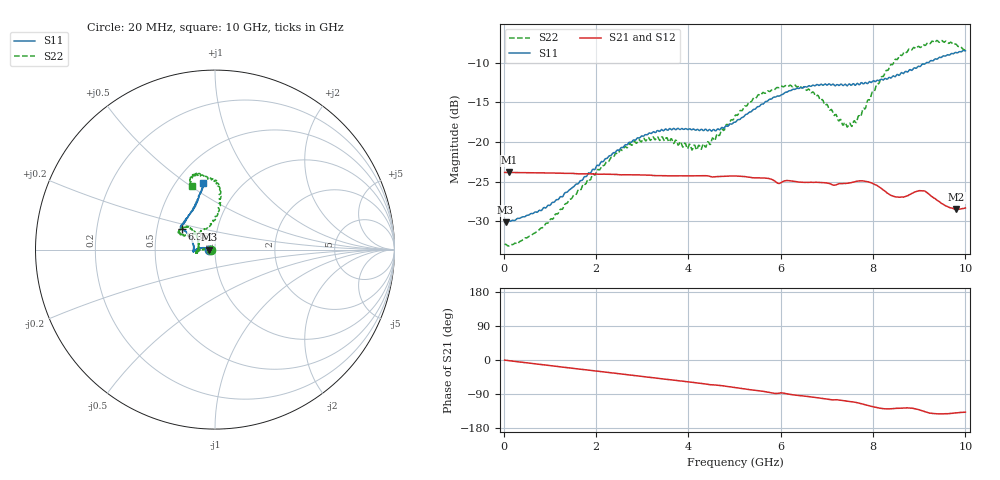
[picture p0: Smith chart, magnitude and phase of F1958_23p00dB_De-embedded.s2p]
! Integrated Device Technology
! Corporate Headquarters
! 6024 Silver Creek Valley Road
! San Jose, CA 95138  USA
! Phone:  1-408-284-8200
! Toll Free:  1-800-223-1366
! Webpage:  http://www.idt.com/
! Timing and RF Division
! 515 Groton Road, Suite 102
! Westford, MA 01886-6024
! Device:  F1958
! Description: 7-bit 0.25 dB Digital Step Attenuator
! Frequency:  0.001 -  6.000 GHz
! Package:  4x4 mm Thin QFN Plastic Package: 24 pin
! Ports:  2 RF, 12 DC
!  Pin  1  = D0
!  Pin  2  = VDD
!  Pin  3  = VMODE
!  Pin  4  = GND
!  Pin  5  = RF1  =  Port 1
!  Pin  6  = GND
!  Pin  7  = GND
!  Pin  8  = GND
!  Pin  9  = GND
!  Pin 10  = GND
!  Pin 11  = GND
!  Pin 12  = GND
!  Pin 13  = GND
!  Pin 14  = RF2  =  Port 2
!  Pin 15  = GND
!  Pin 16  = LE
!  Pin 17  = CLK
!  Pin 18  = DATA
!  Pin 19  = D6
!  Pin 20  = D5
!  Pin 21  = D4
!  Pin 22  = D3
!  Pin 23  = D2
!  Pin 24  = D1
! State:  92
! Atten State:  23.00 dB
! Voltage:  +3.30 Volts
! Current:  0.258 mA
! Data:  The device was measured on a F1958 evaluation board which has
!  individual transmission lines to the RF pins.  Data was collected
!  using a calibrated network analyzer.  The evaluation board was
!  de-embedded using Automatic Fixture Removal (AFR).
!  The reference plane is the edge of the package pin.
! Misc:
!  Action Tracker AT0419
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# GHz S dB R 50
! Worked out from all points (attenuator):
!   500 points, 20 MHz to 10 GHz, reference 50 ohm
!   highest |S21| = -23.84 dB at 120 MHz (marker M1); lowest = -28.5 dB at 9.8 GHz (marker M2)
!   lowest |S11| = -30.1 dB at 40 MHz (marker M3), VSWR 1.06, Z = 47 - j0.0425 ohm
!   |S11| at or under -10 dB: start of sweep to 9.151 GHz
!   |S22| runs from -33.2 to -7.2 dB; largest |S21 - S12| = 0.00036
!   S11 on the Smith chart (normalised r, x): 20 MHz: 0.94, -0.00; 6.36 GHz: 0.67, +0.16; 10 GHz: 0.67, +0.58
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0.02  -30.10 -179.0  -23.85 -0.3  -23.84 -0.3  -32.97 -178.3
0.04  -30.12 -179.2  -23.84 -0.6  -23.84 -0.6  -32.91 -177.5
0.12  -30.01 178.8  -23.84 -1.8  -23.84 -1.8  -33.09 -179.5
0.84  -28.50 170.7  -23.91 -12.4  -23.90 -12.4  -30.83 178.4
1.7  -24.84 170.7  -24.02 -24.7  -24.02 -24.6  -25.62 177.3
2.6  -20.61 176.7  -24.14 -37.6  -24.12 -37.6  -20.83 -177.3
3.36  -18.65 -175.7  -24.25 -48.8  -24.25 -48.9  -19.63 -168.7
4.24  -18.57 -179.0  -24.27 -61.2  -24.28 -61.3  -20.45 169.7
4.52  -18.57 174.0  -24.42 -65.5  -24.43 -65.5  -19.50 154.3
5.02  -17.50 160.7  -24.29 -72.8  -24.31 -72.8  -16.60 139.8
5.58  -15.23 150.5  -24.55 -82.0  -24.56 -81.9  -14.01 140.1
6.36  -13.21 148.2  -25.03 -93.3  -25.05 -93.3  -13.11 153.8
6.68  -12.88 146.7  -25.09 -97.6  -25.11 -97.5  -13.74 155.1
7.32  -12.71 141.5  -25.26 -106.7  -25.27 -106.6  -17.46 135.3
7.5  -12.72 138.4  -25.17 -109.3  -25.17 -109.2  -17.63 117.3
7.68  -12.68 135.5  -24.93 -113.3  -24.93 -113.3  -16.73 99.6
7.9  -12.49 129.1  -25.04 -120.3  -25.03 -120.3  -14.66 89.8
8.34  -11.87 119.1  -26.57 -129.1  -26.57 -129.2  -10.79 83.6
8.82  -10.92 111.6  -26.56 -126.7  -26.57 -126.7  -8.41 90.6
9.12  -10.16 106.7  -26.19 -136.1  -26.20 -136.2  -7.81 98.7
9.8  -8.70 100.8  -28.49 -139.6  -28.52 -139.6  -7.65 109.6
10  -8.49 100.0  -28.33 -137.6  -28.36 -137.8  -8.44 110.2
